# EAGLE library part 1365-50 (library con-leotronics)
DUAL ROW STRAIGHT HEADER 1364 SERIES. 1.27mm x 1.27mm. Without Fixing Post. SMT Source: http://www.leotronics.co.uk/Conexcon/Data%20Sheets/sec.%20A/1364ing.pdf
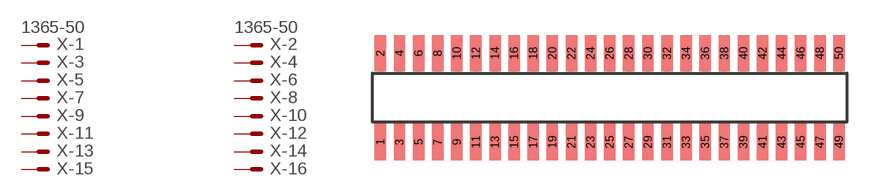
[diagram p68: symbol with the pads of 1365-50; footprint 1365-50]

Designator prefix X; gates -1=MVAL -2=MVAL -3=M -4=M -5=M -6=M -7=M -8=M -9=M -10=M -11=M -12=M -13=M -14=M -15=M -16=M -17=M -18=M -19=M -20=M -21=M -22=M -23=M -24=M -25=M -26=M -27=M -28=M -29=M -30=M -31=M -32=M -33=M -34=M -35=M -36=M -37=M -38=M -39=M -40=M -41=M -42=M -43=M -44=M -45=M -46=M -47=M -48=M -49=M -50=M

## 1365-50 (OC_FARNELL: unknown; OC_NEWARK: unknown)  [1365-50]
1  -1:S  pas
2  -2:S  pas
3  -3:S  pas
4  -4:S  pas
5  -5:S  pas
6  -6:S  pas
7  -7:S  pas
8  -8:S  pas
9  -9:S  pas
10  -10:S  pas
11  -11:S  pas
12  -12:S  pas
13  -13:S  pas
14  -14:S  pas
15  -15:S  pas
16  -16:S  pas
17  -17:S  pas
18  -18:S  pas
19  -19:S  pas
20  -20:S  pas
21  -21:S  pas
22  -22:S  pas
23  -23:S  pas
24  -24:S  pas
25  -25:S  pas
26  -26:S  pas
27  -27:S  pas
28  -28:S  pas
29  -29:S  pas
30  -30:S  pas
31  -31:S  pas
32  -32:S  pas
33  -33:S  pas
34  -34:S  pas
35  -35:S  pas
36  -36:S  pas
37  -37:S  pas
38  -38:S  pas
39  -39:S  pas
40  -40:S  pas
41  -41:S  pas
42  -42:S  pas
43  -43:S  pas
44  -44:S  pas
45  -45:S  pas
46  -46:S  pas
47  -47:S  pas
48  -48:S  pas
49  -49:S  pas
50  -50:S  pas

## Footprint 1365-50 (pad centres in mm)
DUAL ROW STRAIGHT HEADER 1364 SERIES. 1.27mm x 1.27mm. Without Fixing Post. SMT Source: http://www.leotronics.co.uk/Conexcon/Data%20Sheets/sec.%20A/1364ing.pdf
smd 0.76 x 2.4: 1 -15.24,-2.95; 2 -15.24,2.95; 3 -13.97,-2.95; 4 -13.97,2.95; 5 -12.7,-2.95; 6 -12.7,2.95; 7 -11.43,-2.95; 8 -11.43,2.95; 9 -10.16,-2.95; 10 -10.16,2.95; 11 -8.89,-2.95; 12 -8.89,2.95; 13 -7.62,-2.95; 14 -7.62,2.95; 15 -6.35,-2.95; 16 -6.35,2.95; 17 -5.08,-2.95; 18 -5.08,2.95; 19 -3.81,-2.95; 20 -3.81,2.95; 21 -2.54,-2.95; 22 -2.54,2.95; 23 -1.27,-2.95; 24 -1.27,2.95; 25 0,-2.95; 26 0,2.95; 27 1.27,-2.95; 28 1.27,2.95; 29 2.54,-2.95; 30 2.54,2.95; 31 3.81,-2.95; 32 3.81,2.95; 33 5.08,-2.95; 34 5.08,2.95; 35 6.35,-2.95; 36 6.35,2.95; 37 7.62,-2.95; 38 7.62,2.95; 39 8.89,-2.95; 40 8.89,2.95; 41 10.16,-2.95; 42 10.16,2.95; 43 11.43,-2.95; 44 11.43,2.95; 45 12.7,-2.95; 46 12.7,2.95; 47 13.97,-2.95; 48 13.97,2.95; 49 15.24,-2.95; 50 15.24,2.95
